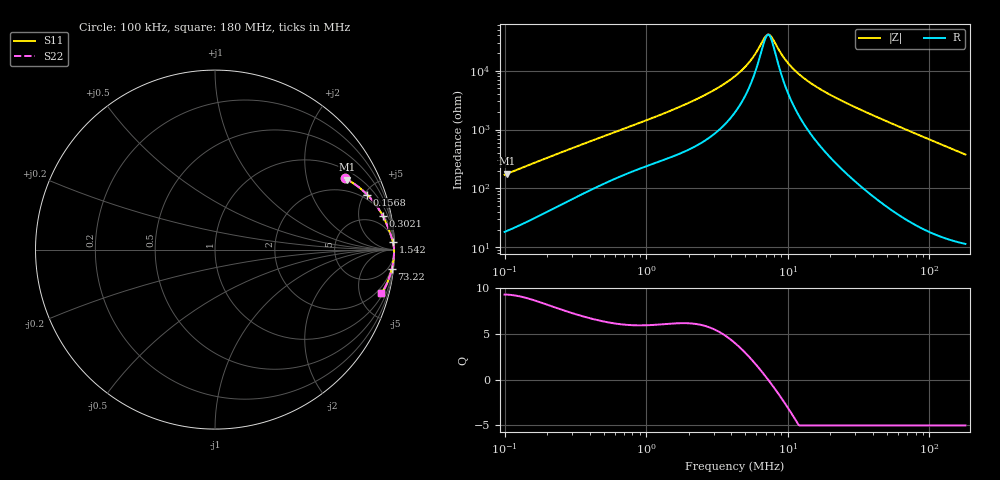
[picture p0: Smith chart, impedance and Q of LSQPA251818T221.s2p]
! LSQPA251818T221  S-PARAMETER MODEL  ( General Type )
! Model Generated by TAIYO YUDEN Corporation (http://www.ty-top.com)
! Version 3.0
! TAIYO YUDEN Control No. 160907NF25SB-FAC
! Copyright(c) 2007 TAIYO YUDEN CO.,LTD. All Rights Reserved.
! Product Description (link to TY-COMPAS)
! https://ds.yuden.co.jp/TYCOMPAS/or/detail?pn=LSQPA251818T221K&u=M
! Products Name : Inductors
! Characteristics :
!  Inductance : 220 uH , SRF(min) : 5.5 MHz , DC Resistance(max) : 10.92 Ohm
!  Rated Current : Saturation :115 mA , Temp Rise : 110 mA (40 degC)
!  Case Size : 2.5 x 1.8 / 0.098 x 0.071 [mm/inch] , Thickness : 1.8 / 0.071 [mm/inch]
!  (Conditions: Temperature = 25 degC , DC Bias Current/Voltage = 0A / 0V)
! External Node Assignments :
!  1  o---GGG---o  2
! GND o---------o GND
! Frequency Range : 0.1MHz  -  180.004543MHz  [ 402 STEP ]
# MHz S RI R 50
! Freq[MHz].  S11 Real  S11 Imag  S21 Real  S21 Imag  S12 Real  S12 Imag  S22 Real  S22 Imag
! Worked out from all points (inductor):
!   401 points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, 100 kHz to 180 MHz, reference 50 ohm
!   read as one part in series: L = 268 uH near 103.8 kHz
!   highest Q = 9.29 at 103.8 kHz (marker M1), where L = 270 uH
!   self-resonance near 7.17 MHz
!   S11 on the Smith chart (normalised r, x): 100 kHz: 1.37, +3.40; 156.8 kHz: 1.60, +5.23; 302.1 kHz: 2.33, +9.62; 1.542 MHz: 8, +43; 73.22 MHz: 2, -19; 180 MHz: 1.23, -7.52
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0.1  0.7238 0.3966  0.2762 -0.3966  0.2762 -0.3966  0.7238 0.3966
0.103819  0.7366 0.39  0.2634 -0.39  0.2634 -0.39  0.7366 0.39
0.15679  0.8476 0.3067  0.1524 -0.3067  0.1524 -0.3067  0.8476 0.3067
0.302102  0.9358 0.1857  0.0642 -0.1857  0.0642 -0.1857  0.9358 0.1857
0.350962  0.9467 0.164  0.0533 -0.164  0.0533 -0.164  0.9467 0.164
1.231743  0.9876 0.0555  0.0124 -0.0555  0.0124 -0.0555  0.9876 0.0555
1.542334  0.9906 0.0448  0.0094 -0.0448  0.0094 -0.0448  0.9906 0.0448
2.86246  0.9955 0.0224  0.00448 -0.0224  0.00448 -0.0224  0.9955 0.0224
4.322947  0.9969 0.0115  0.0031 -0.0115  0.0031 -0.0115  0.9969 0.0115
5.413005  0.9973 0.00636  0.00271 -0.00636  0.00271 -0.00636  0.9973 0.00636
5.944694  0.9974 0.00431  0.00259 -0.00431  0.00259 -0.00431  0.9974 0.00431
6.906137  0.9975 0.0011  0.00246 -0.0011  0.00246 -0.0011  0.9975 0.0011
7.305497  0.9976 -0.000102  0.00242 0.000102  0.00242 0.000102  0.9976 -0.000102
7.727952  0.9976 -0.0013  0.00239 0.0013  0.00239 0.0013  0.9976 -0.0013
9.147624  0.9977 -0.00495  0.00234 0.00495  0.00234 0.00495  0.9977 -0.00495
10.42979  0.9977 -0.00788  0.00233 0.00788  0.00233 0.00788  0.9977 -0.00788
12.11662  0.9976 -0.0114  0.00237 0.0114  0.00237 0.0114  0.9976 -0.0114
14.89024  0.9975 -0.0167  0.00249 0.0167  0.00249 0.0167  0.9975 -0.0167
24.23791  0.9967 -0.0324  0.00329 0.0324  0.00329 0.0324  0.9967 -0.0324
52.25907  0.9917 -0.0749  0.00826 0.0749  0.00826 0.0749  0.9917 -0.0749
73.22333  0.9857 -0.1053  0.0143 0.1053  0.0143 0.1053  0.9857 -0.1053
180.0045  0.9276 -0.2444  0.0724 0.2444  0.0724 0.2444  0.9276 -0.2444
